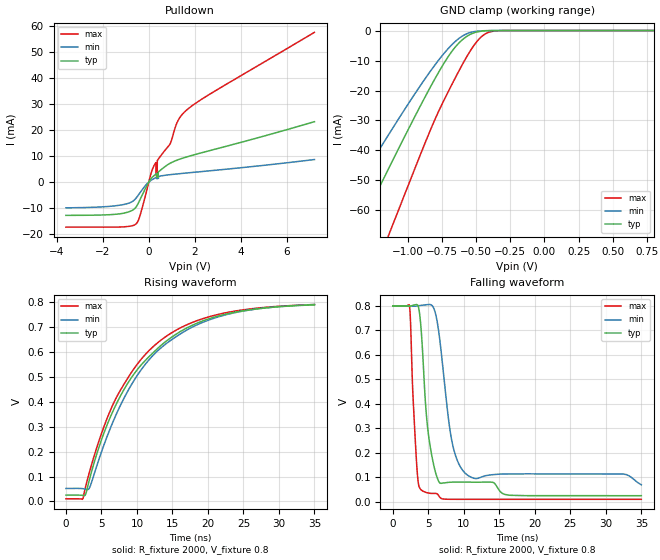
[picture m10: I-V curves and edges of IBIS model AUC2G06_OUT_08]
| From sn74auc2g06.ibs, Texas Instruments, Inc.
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[Model]   AUC2G06_OUT_08
Model_type  Open_drain
Enable   Active-Low
Vref =   0
Rref =   2000
Cref =   15p
Vmeas =   0.4
| variable   typ   min   max
C_comp   3.12pF   2.83pF   3.28pF
| C_pulldown   3.74pF   3.15pF   4.26pF
| C_tri-state   3.12pF   2.83pF   3.28pF
[Temperature Range]   40   100   -40
| Ambient temperature   25   85   -40
[Voltage range]   0.8   0.8   0.8
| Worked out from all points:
|   slope of the pulldown table from 0 to 0.12 V, typ, clamps not added: 77.1 ohm
|   GND clamp passes 1 mA (typ) near -0.53 V on its own axis
|   rising waveform, R_fixture 2000, V_fixture 0.8: 20-80 % time 9.61ns typ, 9.56ns min, 9.01ns max; typ from 0.025 V to 0.791 V
|   falling waveform, R_fixture 2000, V_fixture 0.8: 20-80 % time 1.42ns typ, 1.92ns min, 730ps max; typ from 0.8 V to 0.025 V
[GND Clamp]
| AUC2G06_OUT_08
|   Voltage   I(typ)   I(min)   I(max)
-3.6V     -279.3mA   -228.7mA   -348mA
-1.565V   -85.79mA   -66.64mA   -117.4mA
-1.35V    -65.56mA   -50.29mA   -92.6mA
-1.14V    -46.06mA   -34.73mA   -68.28mA
-1.1V     -42.39mA   -31.84mA   -63.64mA
-830mV    -18.49mA   -13.3mA    -32.72mA
-695mV    -8.11mA    -5.581mA   -19.61mA
-575mV    -2.179mA   -1.221mA   -9.275mA
-505mV    -618.6uA   -292.2uA   -4.307mA
-450mV    -169uA     -82.44uA   -1.67mA
-330mV    -5.484uA   -4.173uA   -50.52uA
800mV     186.8pA    341.4pA    147.7pA
[Pulldown]
| AUC2G06_OUT_08
|   Voltage   I(typ)   I(min)   I(max)
-3.6V     -12.84mA   -9.953mA   -17.38mA
-570mV    -9.824mA   -6.369mA   -16.25mA
-385mV    -6.858mA   -4.174mA   -13.02mA
190mV     2.176mA    1.163mA    5.632mA
310mV     3.079mA    1.693mA    7.502mA
315mV     3.117mA    1.714mA    2.469mA
365mV     1.692mA    1.285mA    2.781mA
370mV     1.723mA    1.302mA    8.254mA
925mV     7.223mA    2.844mA    14.73mA
1.22V     8.419mA    3.123mA    22.74mA
1.49V     9.254mA    3.359mA    26.43mA
7.2V      23.27mA    8.675mA    57.71mA
[Ramp]
| AUC2G06_OUT_08
| variable   typ   min   max
dV/dt_r   0.46/9.61E-09   0.45/9.56E-09   0.47/9.01E-09
dV/dt_f   0.47/1.42E-09   0.44/1.93E-09   0.48/7.33E-10
R_load = 2000
[Rising Waveform]
| AUC2G06_OUT_08
R_fixture =   2000
C_fixture =   0
L_fixture =   0
V_fixture =   0.8
V_fixture_min = 0.8
V_fixture_max = 0.8
|   Time   V(typ)   V(min)   V(max)
0s        25.46mV    52.25mV    10.6mV
2.345ns   24.73mV    51.6mV     9.364mV
2.76ns    28.44mV    48.84mV    58.22mV
3.255ns   82.13mV    52.05mV    112.5mV
5.27ns    269.1mV    221mV      294.3mV
7.59ns    419.7mV    381.6mV    443.6mV
10.32ns   539.8mV    518.5mV    562.2mV
13.26ns   624.3mV    614.6mV    646mV
21.79ns   748.2mV    745mV      754.3mV
34.99ns   790.7mV    791.9mV    791.7mV
[Falling Waveform]
| AUC2G06_OUT_08
R_fixture =   2000
C_fixture =   0
L_fixture =   0
V_fixture =   0.8
V_fixture_min = 0.8
V_fixture_max = 0.8
|   Time   V(typ)   V(min)   V(max)
0s        800mV      800mV      800mV
2.345ns   799.4mV    799.9mV    798.9mV
3.355ns   805.9mV    799.7mV    154.7mV
4.005ns   696.6mV    802.6mV    48.56mV
4.98ns    283.6mV    806mV      36.53mV
5.89ns    134.1mV    781.2mV    34.72mV
6.635ns   76.97mV    657mV      18.28mV
8.36ns    80.72mV    241.9mV    10.69mV
10.52ns   80.92mV    109.5mV    10.6mV
34.99ns   25.47mV    69.84mV    10.6mV
